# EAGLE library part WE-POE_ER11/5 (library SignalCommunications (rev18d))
Power over Ethernet Transformer Characteristics Flyback transformer designed for PoE PDs Input voltage: 36 V to 57 V Switching frequencies: 200–500 kHz Operating temperature: –40 ºC to +125 ºC Insulation test voltage: 1.5 kVAC/1 min Different output powers and voltages available Applications Suitable for PoE IC’s like LTC4267, TPS 23750, TPS 23770, LM5070, LM 5071, LM 5072 Details see: http://katalog.we-online.de/en/pbs/WE-PoE? Updated by Dan Xu 2014-07-08 2014 (C) Wurth Elektronik
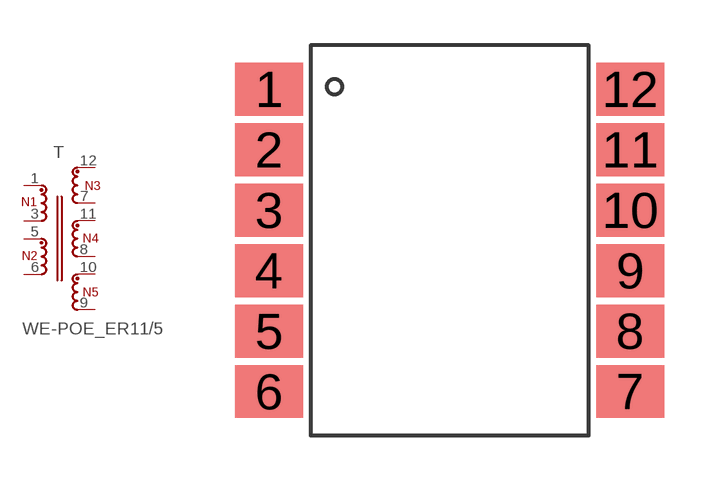
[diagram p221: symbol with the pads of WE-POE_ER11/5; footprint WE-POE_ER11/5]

Designator prefix T

## WE-POE_ER11/5_749119133, WE-POE_ER11/5_749119150  [WE-POE_ER11/5]
1  1  pas
3  2  pas
5  3  pas
6  4  pas
7  6  pas
8  8  pas
9  10  pas
10  9  pas
11  7  pas
12  5  pas

## Footprint WE-POE_ER11/5 (pad centres in mm)
Transformer, ER11/5 SMD 12Pin
smd 2.25 x 1.75: 1 -5.975,5; 2 -5.975,3; 3 -5.975,1; 4 -5.975,-1; 5 -5.975,-3; 6 -5.975,-5; 7 5.975,-5; 8 5.975,-3; 9 5.975,-1; 10 5.975,1; 11 5.975,3; 12 5.975,5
